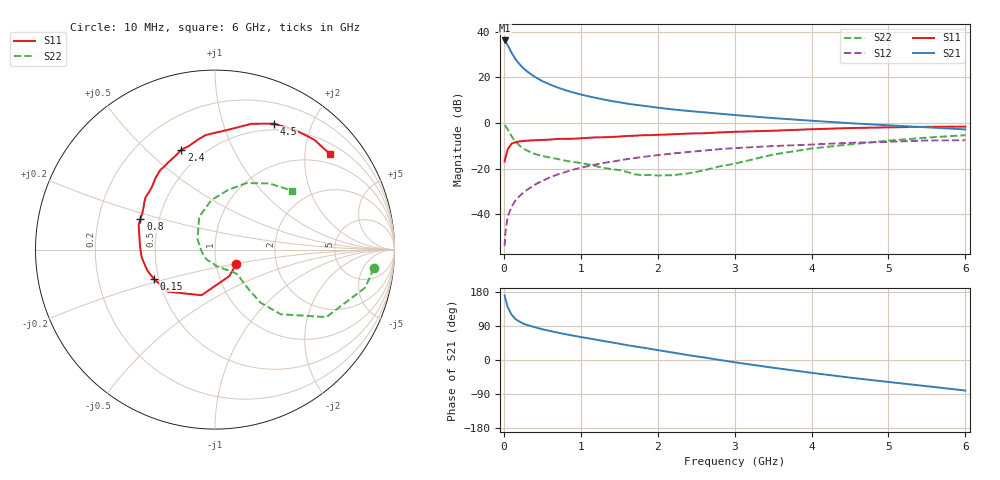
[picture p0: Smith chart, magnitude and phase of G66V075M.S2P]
! SIEMENS Small Signal Semiconductors
! BFG193
! Si NPN RF Bipolar Junction Transistor in SOT223
! VCE = 6 V  IC = 75 mA
! Common Emitter S-Parameters:  August  1996
# GHz  S  MA  R  50
!  f  S11  S21  S12  S22
! GHz  MAG  ANG  MAG  ANG  MAG  ANG  MAG  ANG
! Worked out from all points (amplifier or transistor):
!   36 points, 10 MHz to 6 GHz, reference 50 ohm
!   highest |S21| = 36.2 dB at 10 MHz (marker M1)
!   |S21| within 3 dB of that: start of sweep to 64.4 MHz
!   unconditionally stable (mu >= 1): 353.3 MHz to 2.378 GHz
!   at 250 MHz: K = 0.95, MSG = 27.4 dB, |S12| = -30.6 dB
!   at 1.4 GHz: K = 1.05, MAG = 11.9 dB, |S12| = -17.0 dB
!   at 6 GHz: K = 0.90, MSG = 2.4 dB, |S12| = -7.5 dB
!   S11 on the Smith chart (normalised r, x): 10 MHz: 1.25, -0.21; 150 MHz: 0.47, -0.18; 800 MHz: 0.39, +0.17; 2.4 GHz: 0.38, +0.65; 4.5 GHz: 0.42, +1.49; 6 GHz: 0.74, +2.58
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0.01  0.143 -34.3  64.33 170.2  0.002 81.7  0.8914 -6.7
0.02  0.1682 -61.8  61.81 161.7  0.0039 78.3  0.8632 -14.2
0.05  0.2652 -106.5  50.76 139.9  0.0088 71.4  0.7257 -31.2
0.1  0.3517 -138.2  34.83 119.9  0.0147 68.8  0.5142 -44.5
0.15  0.3778 -154.6  25.22 108.1  0.0199 68.5  0.3911 -49.3
0.2  0.3938 -162.5  19.74 101.7  0.0245 69.9  0.3249 -49.6
0.25  0.4029 -169.5  16.08 96.4  0.0294 70.1  0.2764 -49.6
0.3  0.4108 -174.3  13.55 92.5  0.0341 71.1  0.2498 -49.6
0.4  0.418 177.9  10.32 86.7  0.0443 71.0  0.2107 -48.4
0.5  0.4249 171.7  8.275 81.1  0.0539 70.3  0.1886 -47.9
0.6  0.4337 167.1  6.954 76.6  0.0646 68.8  0.1751 -48.9
0.7  0.4469 162.1  5.987 72.2  0.0745 67.5  0.1624 -51.1
0.8  0.4497 157.7  5.232 68.1  0.0842 65.4  0.1497 -52.9
1.1  0.4737 146.3  3.845 57.2  0.1141 60.3  0.1238 -63.5
1.3  0.4869 139.7  3.264 50.0  0.1335 56.2  0.1037 -71.2
1.6  0.5196 129.5  2.659 39.2  0.1617 49.3  0.0849 -91.6
2.2  0.5658 113.1  1.98 19.5  0.2153 35.7  0.072 -153.7
2.4  0.587 108.7  1.835 12.7  0.2319 31.4  0.0787 178.9
3.5  0.6762 82.7  1.279 -20.4  0.3122 4.3  0.2032 115.7
4.5  0.7745 65.0  0.989 -46.5  0.368 -15.8  0.3394 77.8
5.5  0.825 48.0  0.804 -69.2  0.4138 -39.4  0.4778 50.5
6  0.8328 39.7  0.723 -80.6  0.4195 -52.9  0.5398 37.4
